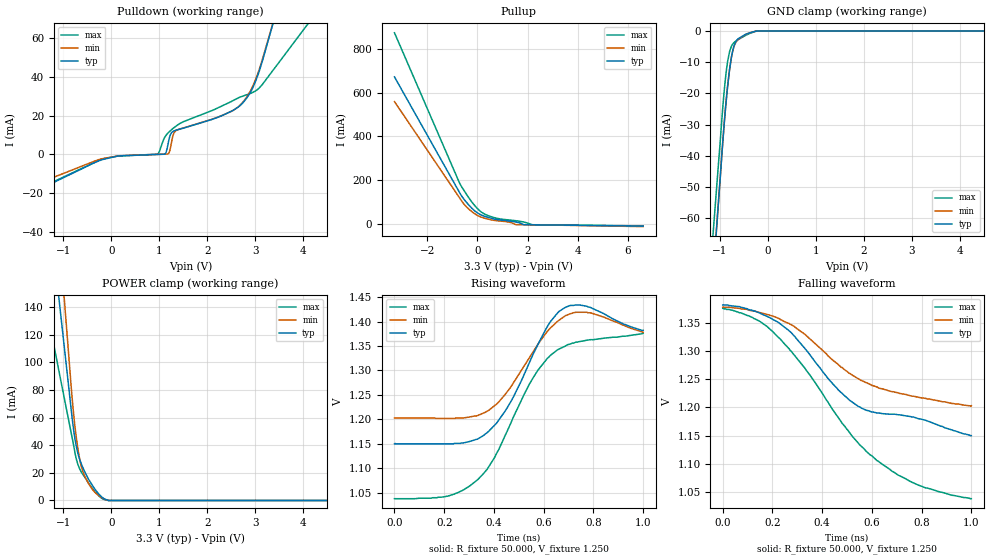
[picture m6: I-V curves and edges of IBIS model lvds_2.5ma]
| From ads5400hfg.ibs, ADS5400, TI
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[Model]   lvds_2.5ma
Model_type 3-state
Vref=1.250E+00
Rref=5.000E+01
Cref=0.000E+00
Vmeas=1.250E+00
C_comp   4.960E-13   4.830E-13   5.040E-13
[Voltage Range]   3.300E+00   3.000E+00   3.600E+00
[POWER Clamp Reference]   3.300E+00   3.000E+00   3.600E+00
[GND Clamp Reference]   0.000E+00   0.000E+00   0.000E+00
[Pullup Reference]   3.300E+00   3.000E+00   3.600E+00
[Pulldown Reference]   0.000E+00   0.000E+00   0.000E+00
[Temperature Range]   25   100   -40
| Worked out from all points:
|   slope of the pulldown table from 0 to 0.495 V, typ, clamps not added: 430 ohm
|   slope of the pullup table from 0 to 0.495 V, typ, clamps not added: 21.5 ohm
|   GND clamp passes 1 mA (typ) near -0.45 V on its own axis
|   POWER clamp passes 1 mA (typ) near -0.14 V on its own axis
|   rising waveform, R_fixture 50.000, V_fixture 1.250: 20-80 % time 143ps typ, 140ps min, 207ps max; typ from 1.15 V to 1.38 V
|   falling waveform, R_fixture 50.000, V_fixture 1.250: 20-80 % time 302ps typ, 319ps min, 363ps max; typ from 1.38 V to 1.15 V
[GND Clamp]
-3.3V     -539mA     -540.7mA   -496.2mA
-1.02V    -52.83mA   -52.82mA   -40.7mA
-940mV    -35.68mA   -35.61mA   -24.58mA
-880mV    -24.35mA   -24.22mA   -14.67mA
-840mV    -17.94mA   -17.84mA   -9.882mA
-800mV    -12.57mA   -12.53mA   -6.72mA
-760mV    -8.428mA   -8.477mA   -4.915mA
-720mV    -5.548mA   -5.691mA   -3.947mA
-660mV    -3.23mA    -3.455mA   -3.162mA
-440mV    -923.3uA   -991uA     -1.218mA
-220mV    0A         0A         0A
6.6V      0A         0A         0A
[Power Clamp]
-3.3V     841.4mA    1.162A     481mA
-900mV    85.31mA    109.9mA    59.72mA
-820mV    60.16mA    74.86mA    45.68mA
-760mV    44.68mA    53.54mA    34.71mA
-700mV    34.32mA    37.9mA     26.3mA
-640mV    27.64mA    26.55mA    21.43mA
-560mV    21.11mA    17.8mA     17.13mA
-420mV    12.27mA    9.225mA    9.853mA
-320mV    7.109mA    5.101mA    5.439mA
-180mV    1.972mA    1.595mA    1.137mA
-60mV     0A         0A         0A
6.6V      0A         0A         0A
[Pullup]
-3.3V     671.5mA    558.8mA    872.6mA
-700mV    142.4mA    118.5mA    185.6mA
-560mV    118.1mA    95.28mA    158.9mA
-340mV    87.33mA    68.63mA    120.5mA
-60mV     56.77mA    44.25mA    79.17mA
140mV     42.77mA    32.84mA    56.89mA
680mV     23.35mA    17.17mA    29.71mA
1.32V     13.91mA    7.97mA     18.54mA
1.54V     9.933mA    -2.14mA    15.59mA
1.86V     -2.295mA   -2.823mA   9.58mA
2.2V      -2.956mA   -3.17mA    -2.48mA
6.6V      -8.999mA   -10.97mA   -7.89mA
[Pulldown]
-3.3V     -39.67mA   -32.37mA   -38.55mA
-260mV    -3.285mA   -2.641mA   -3.037mA
960mV     -4.036uA   30.85uA    141.4uA
1.12V     280.5uA    169.3uA    9.192mA
1.18V     5.319mA    279.2uA    11.08mA
1.24V     10.73mA    4.465mA    12.5mA
1.34V     12.46mA    12.29mA    14.5mA
2.28V     19.79mA    19.87mA    24.76mA
2.72V     26.13mA    26.42mA    29.96mA
2.94V     34.11mA    34.92mA    31.97mA
3.16V     49.38mA    50.18mA    36.58mA
6.6V      349.9mA    344.5mA    150mA
[Rising Waveform]
R_fixture = 50.000
V_fixture = 1.250
V_fixture_min = 1.250
V_fixture_max = 1.250
|  time   V(typ)   V(min)   V(max)
0s        1.15V      1.203V     1.038V
240ps     1.151V     1.202V     1.047V
302.5ps   1.155V     1.205V     1.064V
377.5ps   1.175V     1.218V     1.102V
467.5ps   1.236V     1.266V     1.192V
562.5ps   1.338V     1.342V     1.289V
627.5ps   1.4V       1.387V     1.331V
687.5ps   1.429V     1.412V     1.35V
787.5ps   1.429V     1.418V     1.363V
1ns       1.382V     1.378V     1.376V
[Falling Waveform]
R_fixture = 50.000
V_fixture = 1.250
V_fixture_min = 1.250
V_fixture_max = 1.250
|  time   V(typ)   V(min)   V(max)
0s        1.382V     1.378V     1.376V
152.5ps   1.367V     1.368V     1.352V
232.5ps   1.348V     1.356V     1.321V
275ps     1.333V     1.347V     1.3V
330ps     1.305V     1.33V      1.27V
465ps     1.231V     1.276V     1.182V
545ps     1.202V     1.251V     1.137V
622.5ps   1.19V      1.236V     1.105V
787.5ps   1.18V      1.218V     1.062V
1ns       1.15V      1.203V     1.038V
[Ramp]
dV/dt_f   1.3920E-01/6.0066E-10   1.0500E-01/3.3469E-10   2.0280E-01/4.0828E-10
dV/dt_r   1.3920E-01/1.5070E-10   1.0500E-01/1.4700E-10   2.0280E-01/2.2600E-10
R_load = 50
